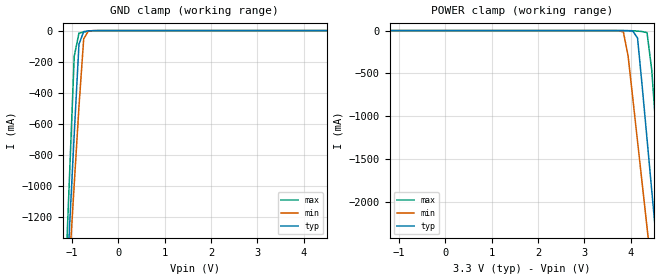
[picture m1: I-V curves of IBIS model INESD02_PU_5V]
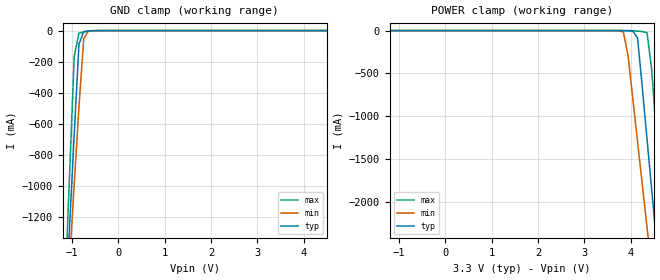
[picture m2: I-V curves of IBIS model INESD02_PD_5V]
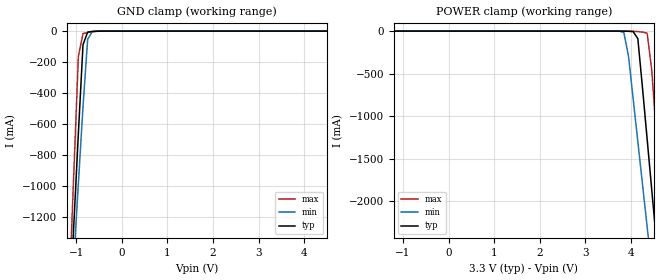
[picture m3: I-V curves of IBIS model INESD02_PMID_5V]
|   This file is an IBIS representation of the   |
|   Integrated Device Technology, Inc   |
|   ICS854104I   |
|   LOW SKEW, 1-TO-4 DIFFERENTIAL-TO-LVDS FANOUT BUFFER   |
[IBIS Ver]   4.1
[File name]   854104i_3v3.ibs
[File Rev]   1.0
[Date]   9 Mar 2010
[Source]   Originated at Integrated Device Technology, Inc.
[Disclaimer]
IDT hereby grants the user of this IBIS model a non-exclusive,
nontransferable license to use this IBIS model under the following terms.
Before using this IBIS model, the user should read this license.
If the user does not accept these terms,  the IBIS model should be
returned to IDT within 30 days.
   The user is granted this license only to use the IBIS model and
is not granted rights to sell, load, rent, lease or license the IBIS
model in whole or in part, or in modified form to anyone other than
user. User may modify the IBIS model to suit its specific
applications but rights to derivative works and such modifications
shall belong to IDT.
   This IBIS model is provided on an "AS IS" basis and IDT makes
absolutely no warranty with respect to the information contained
herein. IDT DISCLAIMS AND CUSTOMER WAIVES ALL WARRANTIES, EXPRESS
OR IMPLIED, INCLUDING WARRANTIES OF MERCHANTABILITY OR FITNESS FOR
A PARTICULAR PURPOSE. The entire risk as to quality and performance
is with the Customer. ACCORDINGLY, IN NO EVENT SHALL THE COMPANY BE
LIABLE FOR ANY DAMAGES, WHETHER IN CONTRACT OR TORT,INCLUDING ANY
LOST PROFITS OR OTHER INCIDENTAL, CONSEQUENTIAL, EXEMPLARY, OR
PUNITIVE DAMAGES ARISING OUT OF THE USE OR APPLICATION OF THE IBIS
model provided in this package. Further, IDT reserves the right to
make changes without notice to any product herein to improve
reliability, function, or design. IDT does not convey any license
under patent rights or any other intellectual property rights,
including those of third parties.
   IDT is not obligated to provide maintenance or support
for the licensed IBIS model.
[Copyright]   Copyright 2010 by Integrated Device Technology, Inc.
[Component]   ICS854104AGI
[Manufacturer] Integrated Device Technology, Inc.
[Package]
|   TSSOP16   typ   min   max
R_pkg   58.65m   52.5m   64.8m
L_pkg   1.902nH   1.443nH   2.361nH
C_pkg   0.315pF   0.254pF   0.375pF
[Pin] signal_name   model_name   R_pin   L_pin   C_pin
1  OE0   INESD02_PU_5V   64.8m   2.361n   0.375p
2  OE1   INESD02_PU_5V   60.7m   2.054n   0.335p
3  OE2   INESD02_PU_5V   56.6m   1.749n   0.294p
4  VDD   POWER   52.5m   1.443n   0.254p
5  GND   GND   52.5m   1.443n   0.254p
6  CLK   INESD02_PD_5V   56.6m   1.749n   0.294p
7  nCLK   INESD02_PMID_5V   60.7m   2.054n   0.335p
8  OE3   INESD02_PU_5V   64.8m   2.361n   0.375p
9  nQ3   ONLVDS07_LVDS02_   64.8m   2.361n   0.375p
10 Q3   ONLVDS07_LVDS02_   60.7m   2.054n   0.335p
11 nQ2   ONLVDS07_LVDS02_   56.6m   1.749n   0.294p
12 Q2   ONLVDS07_LVDS02_   52.5m   1.443n   0.254p
13 nQ1   ONLVDS07_LVDS02_   52.5m   1.443n   0.254p
14 Q1   ONLVDS07_LVDS02_   56.6m   1.749n   0.294p
15 nQ0   ONLVDS07_LVDS02_   60.7m   2.054n   0.335p
16 Q0   ONLVDS07_LVDS02_   64.8m   2.361n   0.375p
[Diff Pin]  inv_pin  vdiff tdelay_typ tdelay_min  tdelay_max
6   7   0.15   0   0   0
10   9   NA   0   0   0
12   11   NA   0   0   0
14   13   NA   0   0   0
16   15   NA   0   0   0
| Models and submodels in the file (4): INESD02_PU_5V (Input), INESD02_PD_5V (Input), INESD02_PMID_5V (Input), ONLVDS07_LVDS02_ (Output)
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[Model]   INESD02_PU_5V
Model_type   Input
Polarity   Non-Inverting
Vinl = 0.8V
Vinh = 2.0V
|   typ   min   max
C_comp   2pF   1.5pF   2.5pF
|   typ   min   max
[Voltage range]  3.3V   3.135V   3.465V
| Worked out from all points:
|   GND clamp passes 1 mA (typ) near -0.58 V on its own axis
[GND_clamp]
|Voltage   I(typ)   I(min)   I(max)
-3.3V     -14.52A    -12.53A    -17.87A
-1.157V   -1.867A    -1.989A    -1.704A
-1.055V   -1.265A    -1.488A    -934.1mA
-952.6mV  -663.5mA   -987.5mA   -164.6mA
-850.5mV  -87.67mA   -487.6mA   -16.09mA
-748.5mV  -6.381mA   -52.8mA    -9.221mA
-646.4mV  -1.974mA   -2.739mA   -4.198mA
-340.2mV  -74.07uA   -86.47uA   -63.25uA
6.6V      64.29uA    84.42uA    47.33uA
[POWER_clamp]
|Voltage   I(typ)   I(min)   I(max)
-3.3V     64.29uA    80.4uA     49.82uA
3.64V     -74.07uA   -182uA     -54.96uA
3.844V    -481.8uA   -15.93mA   -77.98uA
3.946V    -1.974mA   -296.1mA   -341uA
4.048V    -6.381mA   -795.8mA   -1.985mA
4.151V    -87.67mA   -1.296A    -5.959mA
4.355V    -1.265A    -2.297A    -23.88mA
4.457V    -1.867A    -2.799A    -459.4mA
4.559V    -2.47A     -3.3A      -1.229A
4.661V    -3.072A    -3.801A    -1.999A
4.763V    -3.675A    -4.303A    -2.769A
6.6V      -14.52A    -13.34A    -16.63A
[Model]   INESD02_PD_5V
Model_type  Input
Polarity   Non-Inverting
Vinl = 0.8V
Vinh = 2.0V
|   typ   min   max
C_comp   2pF   1.5pF   2.5pF
|   typ   min   max
[Voltage range]  3.3V   3.15V   3.45V
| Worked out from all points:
|   GND clamp passes 1 mA (typ) near -0.58 V on its own axis
[GND_clamp]
|Voltage   I(typ)   I(min)   I(max)
-1.973V   -6.688A    -6A        -7.863A
-1.157V   -1.867A    -1.988A    -1.704A
-1.055V   -1.265A    -1.488A    -934.1mA
-952.6mV  -663.4mA   -987.4mA   -164.5mA
-850.5mV  -87.6mA    -487.5mA   -16.04mA
-748.5mV  -6.317mA   -52.72mA   -9.171mA
-646.4mV  -1.91mA    -2.66mA    -4.148mA
-340.2mV  -9.776uA   -8.593uA   -12.08uA
6.6V      128.6uA    131.6uA    121.8uA
[POWER_clamp]
|Voltage   I(typ)   I(min)   I(max)
-3.3V     128.6uA    128.3uA    124.8uA
3.64V     -9.776uA   -103.4uA   -3.241uA
3.844V    -417.5uA   -15.85mA   -26.94uA
3.946V    -1.91mA    -296.1mA   -290.3uA
4.048V    -6.317mA   -795.7mA   -1.934mA
4.151V    -87.6mA    -1.296A    -5.908mA
4.355V    -1.265A    -2.297A    -23.83mA
4.457V    -1.867A    -2.799A    -459.4mA
4.559V    -2.47A     -3.3A      -1.229A
4.661V    -3.072A    -3.801A    -1.999A
4.763V    -3.675A    -4.303A    -2.769A
5.681V    -9.099A    -8.82A     -9.698A
[Model]   INESD02_PMID_5V
Model_type   Input
Polarity   Non-Inverting
Vinl = .8V
Vinh =  2V
|   typ   min   max
C_comp   2pF   1.5pF   2.5pF
|   typ   min   max
[Voltage range]  3.3V   3.15V   3.45V
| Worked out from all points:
|   GND clamp passes 1 mA (typ) near -0.58 V on its own axis
[GND_clamp]
|Voltage   I(typ)   I(min)   I(max)
-3.3V     -14.52A    -12.53A    -17.87A
-1.157V   -1.867A    -1.989A    -1.704A
-1.055V   -1.265A    -1.488A    -934.2mA
-952.6mV  -663.5mA   -987.5mA   -164.6mA
-850.5mV  -87.69mA   -487.6mA   -16.11mA
-748.5mV  -6.402mA   -52.83mA   -9.238mA
-646.4mV  -1.994mA   -2.763mA   -4.213mA
-340.2mV  -86.57uA   -101.8uA   -73.13uA
6.6V      207.5uA    263.8uA    158.1uA
[POWER_clamp]
|Voltage   I(typ)   I(min)   I(max)
-3.3V     207.5uA    255.1uA    163.5uA
3.64V     -86.57uA   -202uA     -61.97uA
3.844V    -498.9uA   -15.95mA   -88.54uA
3.946V    -1.994mA   -296.2mA   -353.3uA
4.048V    -6.402mA   -795.8mA   -1.999mA
4.151V    -87.69mA   -1.296A    -5.974mA
4.355V    -1.265A    -2.297A    -23.9mA
4.457V    -1.867A    -2.799A    -459.5mA
4.559V    -2.47A     -3.3A      -1.229A
4.661V    -3.072A    -3.801A    -1.999A
4.763V    -3.675A    -4.303A    -2.769A
6.6V      -14.52A    -13.34A    -16.63A
